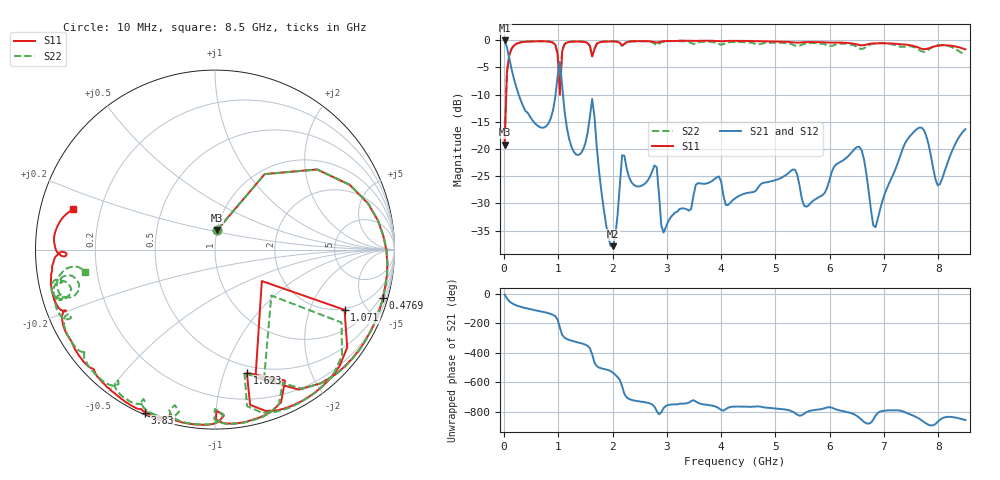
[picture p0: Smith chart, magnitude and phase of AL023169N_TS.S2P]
!AVX CORPORATION
!PN: AL023169N_TS
!DESCRIPTION: AIR CORE INDUCTOR, 169nH, 12 Turns
!Agilent Technologies,E5071C,MY46102230,A.09.54
!Date: Mon Sep 03 16:45:26 2012
!Data & Calibration Information:
!Freq	S11:SOLT2(ON)	S21:SOLT2(ON)	S12:SOLT2(ON)	S22:SOLT2(ON)
# Hz S dB R 50
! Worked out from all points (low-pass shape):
!   201 points, 10 MHz to 8.5 GHz, reference 50 ohm
!   highest |S21| = -0.05 dB at 10 MHz (marker M1); lowest = -37.9 dB at 2.005 GHz (marker M2)
!   |S21| within 3 dB of the highest: start of sweep to 89.72 MHz
!   lowest |S11| = -19.2 dB at 10 MHz (marker M3), VSWR 1.25, Z = 50 + j11 ohm
!   |S11| at or under -10 dB: start of sweep to 39.51 MHz; 1.028484 GHz to 1.029095 GHz (611.6 kHz wide, 0.0595 % of centre)
!   |S22| runs from -19.1 to -0.2 dB; largest |S21 - S12| = 0.0098
!   S11 on the Smith chart (normalised r, x): 10 MHz: 1.00, +0.22; 476.9 MHz: 0.69, -7.05; 1.071 GHz: 1.93, -3.53; 1.623 GHz: 0.43, -1.20; 3.83 GHz: 0.01, -0.66; 8.5 GHz: 0.10, +0.14
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1e7  -19.21 83.6  -0.05 -6.9  -0.04 -7.4  -19.12 83.7
9.49e7  -2.82 38.2  -3.29 -51.6  -3.28 -51.6  -2.80 38.0
4.7695e8  -0.23 -16.0  -14.04 -105.5  -14.03 -105.7  -0.22 -16.5
8.1655e8  -0.25 -42.4  -15.32 -132.8  -15.32 -132.9  -0.22 -42.5
9.8635e8  -2.53 -72.4  -6.64 -175.8  -6.64 -175.8  -2.31 -69.0
1.0288e9  -10.06 -33.9  -3.98 128.6  -3.97 128.5  -7.86 -39.2
1.07125e9  -1.98 -24.9  -8.53 80.3  -8.53 80.3  -1.79 -30.0
1.4533e9  -0.29 -65.9  -20.19 20.1  -20.20 19.9  -0.26 -67.3
1.6231e9  -2.98 -75.5  -10.80 -51.1  -10.80 -51.2  -2.96 -76.6
2.00515e9  -0.22 -83.4  -37.88 -174.8  -37.93 -175.1  -0.22 -84.1
2.17495e9  -0.96 -89.5  -21.14 93.4  -21.16 93.4  -1.03 -90.1
2.85415e9  -0.34 -105.1  -28.25 -96.6  -28.27 -96.5  -0.67 -102.5
2.93905e9  -0.18 -107.4  -35.38 -55.2  -35.41 -55.0  -0.26 -105.2
3.8305e9  -0.10 -113.2  -25.90 -38.1  -25.89 -38.2  -0.32 -123.4
4.255e9  -0.12 -117.7  -29.11 -44.6  -29.11 -44.7  -0.34 -131.7
5.6983e9  -0.35 -140.8  -29.48 -68.9  -29.51 -69.0  -0.52 -159.5
6.50485e9  -0.78 -157.6  -19.62 -108.9  -19.62 -108.9  -1.27 -168.4
6.802e9  -0.60 -160.6  -34.04 -133.6  -34.07 -133.8  -0.65 -163.6
7.09915e9  -0.58 -167.6  -26.21 -70.3  -26.24 -70.2  -0.67 -168.4
7.651e9  -1.40 -179.2  -16.08 -127.2  -16.08 -127.3  -1.83 -169.7
8.03305e9  -0.97 178.2  -26.44 -133.1  -26.48 -133.5  -0.88 -165.6
8.5e9  -1.68 164.2  -16.37 -135.8  -16.38 -135.9  -2.66 -170.4
